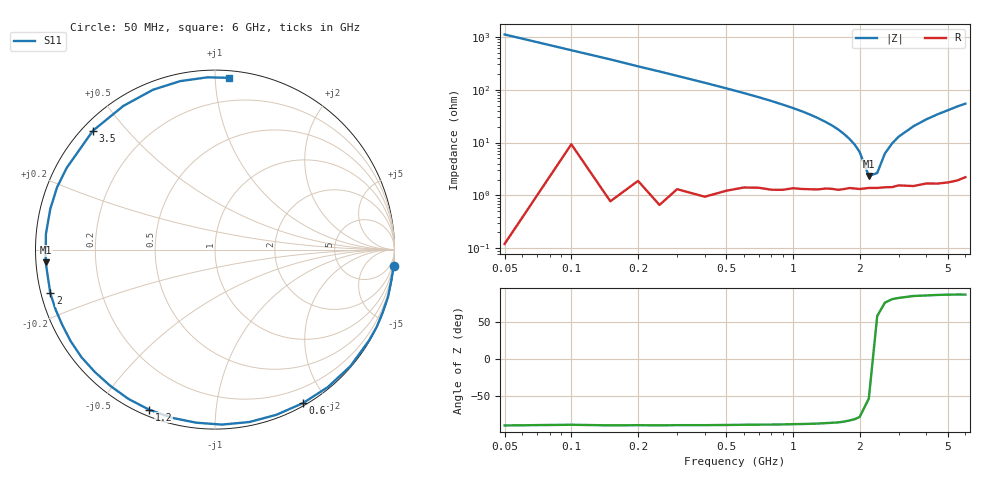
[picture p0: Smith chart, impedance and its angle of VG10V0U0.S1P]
! Infineon Technologies  Discrete & RF Semiconductors
! BB 831
! Si Tuning Diode in SOD323
! VR = 10 V
! S-Parameters:  July  1999
# GHz  S  MA  R  50
!  f  S11
! GHz  MAG  ANG
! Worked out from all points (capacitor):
!   34 points, 50 MHz to 6 GHz, reference 50 ohm
!   read as one part to ground: C = 2.86 pF near 50 MHz
!   lowest |Z| = 2.33 ohm at 2.2 GHz (marker M1)
!   series resonance near 2.291 GHz, so ESL is about 1.7 nH
!   S11 on the Smith chart (normalised r, x): 50 MHz: 0, -22; 600 MHz: 0.03, -1.72; 1.2 GHz: 0.03, -0.67; 2 GHz: 0.03, -0.13; 3.5 GHz: 0.03, +0.41; 6 GHz: 0.04, +1.08
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0.05  1 -5.2
0.15  0.9994 -15.3
0.25  0.9987 -25.6
0.3  0.9963 -30.7
0.4  0.9954 -40.7
0.5  0.9911 -50.6
0.6  0.9859 -60.2
0.7  0.9819 -69.6
0.8  0.9796 -78.7
0.9  0.9758 -87.7
1  0.9701 -96.2
1.1  0.9674 -104.4
1.2  0.9644 -112.4
1.4  0.9574 -127.5
1.6  0.9556 -141.1
1.8  0.9489 -153.8
2  0.9493 -165.2
2.2  0.9461 -175.7
2.4  0.9461 174.8
2.6  0.9452 166.2
2.8  0.946 158.5
3  0.9435 151.2
3.5  0.9495 135.8
4  0.9495 122.5
4.5  0.9553 111.2
5  0.9585 101.7
5.5  0.9608 92.5
6  0.9601 85.3
